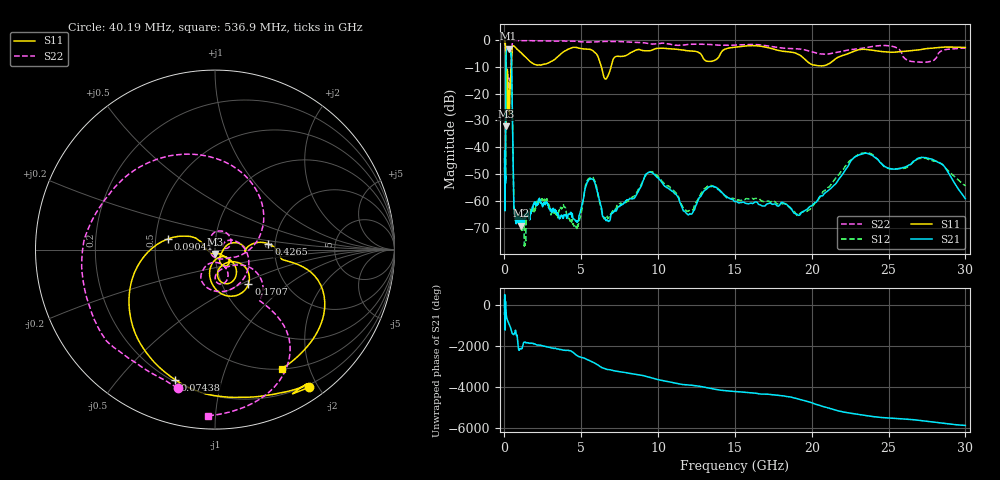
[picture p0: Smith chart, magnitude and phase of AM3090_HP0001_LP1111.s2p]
! Date/Time: Thu, Feb 28, 2019 1:54 PM
! Network Analyzer: Agilent Technologies E8364B Rev: A.07.50.67
! Sweep from 0.010 to 30.000 GHz, 1601 Points, Sweep Type: LOG
! Power Supply: 5.022 V, 0.002 A
# Hz S DB R 50
!freq MagS11 AngS11 MagS21 AngS21 MagS12 AngS12 MagS22 AngS22
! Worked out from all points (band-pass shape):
!   1601 points, 10 MHz to 30 GHz, reference 50 ohm
!   highest |S21| = -3.30 dB at 265.1 MHz (marker M1); lowest = -69.2 dB at 1.066 GHz (marker M2)
!   |S21| within 3 dB of the highest: 102.2 MHz to 441.4 MHz (339.2 MHz wide, 125 % of centre)
!   lowest |S11| = -32.2 dB at 98.93 MHz (marker M3), VSWR 1.05, Z = 49.9 - j2.44 ohm
!   |S11| at or under -10 dB: 89.63 MHz to 429.4 MHz (339.8 MHz wide, 131 % of centre); 6.308 GHz to 6.937 GHz (628.6 MHz wide, 9.49 % of centre)
!   |S22| runs from -31.7 to -0.2 dB; largest |S21 - S12| = 0.0099
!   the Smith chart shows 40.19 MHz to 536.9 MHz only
!   S11 on the Smith chart (normalised r, x): 40.19 MHz: 0.17, -1.89; 74.38 MHz: 0.21, -0.72; 90.41 MHz: 0.58, +0.07; 170.7 MHz: 1.33, -0.55; 426.5 MHz: 1.84, +0.13; 536.9 MHz: 0.50, -1.59
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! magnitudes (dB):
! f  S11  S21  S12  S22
! 10 MHz  -0.2  -41.3  -44.1  -0.7
! 38.04 MHz  -0.5  -63.5  -59.6  -1.8
! 40.19 MHz  -0.6  -62.7  -59.9  -2.0
! 74.38 MHz  -2.4  -46.0  -46.3  -4.2
! 90.41 MHz  -11.4  -14.8  -14.8  -12.6
! 98.93 MHz  -32.2  -7.2  -7.2  -31.6
! 113.2 MHz  -14.2  -4.9  -4.9  -19.5
! 144.7 MHz  -18.7  -3.6  -3.6  -24.5
! 170.7 MHz  -11.5  -3.5  -3.4  -14.4
! 265.1 MHz  -21.1  -3.3  -3.3  -17.4
! 426.5 MHz  -10.5  -5.4  -5.4  -10.6
! 536.9 MHz  -2.4  -38.1  -37.9  -0.7
! 550.5 MHz  -2.3  -42.7  -42.6  -0.5
! 646.1 MHz  -2.4  -63.8  -64.9  -0.2
! 1.066 GHz  -4.7  -69.2  -68.3  -0.3
! 1.341 GHz  -6.2  -65.9  -76.1  -0.3
! 2.084 GHz  -9.4  -61.3  -60.8  -0.3
! 7.926 GHz  -5.8  -59.8  -60.5  -0.8
! 9.586 GHz  -3.8  -49.4  -49.1  -1.6
! 19.31 GHz  -6.0  -64.4  -64.2  -3.4
! 23.48 GHz  -3.5  -42.2  -42.0  -2.9
! 30 GHz  -2.8  -59.1  -54.4  -3.1
